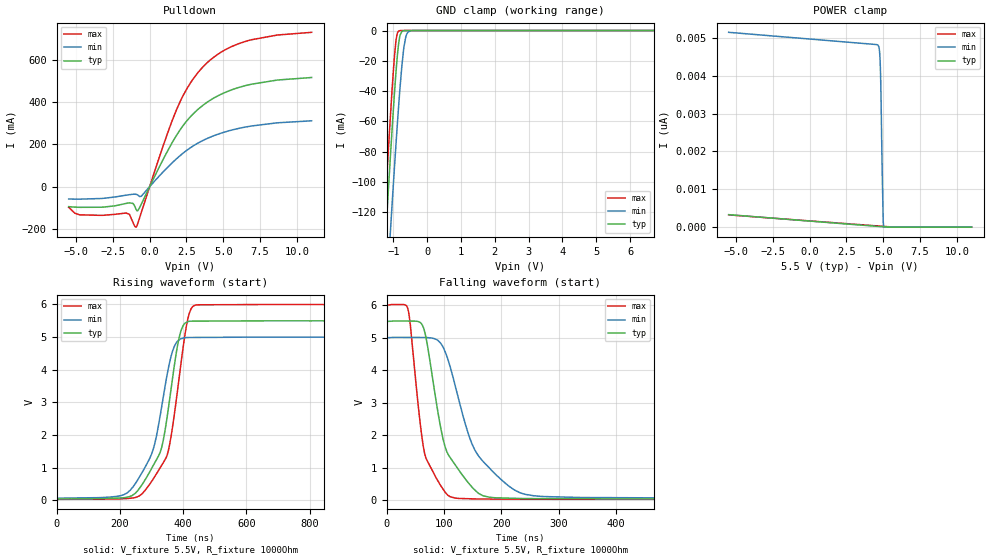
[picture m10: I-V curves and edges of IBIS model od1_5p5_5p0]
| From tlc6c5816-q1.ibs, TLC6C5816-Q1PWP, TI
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|   od1_5p5_5p0 Model
[Model]   od1_5p5_5p0
Model_type   Open_drain
Polarity   Inverting
Vmeas = 2.75
Vref = 5.5
Cref = 2pF
Rref = 1000
|   typ   min   max
C_comp   4.463pF   3.923pF   4.609pF
| Where Nom  PVT is Nominal Process, 5.5V, 27C
|   Fast PVT is Strong Process,  6.0V, -40C
|   Slow PVT is Weak Process,   5.0V, 150C
[Voltage Range]   5.5   5   6
|Junction Temperature
[Temperature Range]   27   150   -40
[Pullup Reference]   5.5   5   6
[Pulldown Reference]   0   -0   0
[Power Clamp Reference]   5.5   5   6
[GND Clamp Reference]   0   0   0
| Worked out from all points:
|   slope of the pulldown table from 0 to 0.825 V, typ, clamps not added: 7.09 ohm
|   GND clamp passes 1 mA (typ) near -0.76 V on its own axis
|   falling waveform, V_fixture 5.5V, R_fixture 1000Ohm: 20-80 % time 43.5ns typ, 63.8ns min, 26ns max; typ from 5.5 V to 0.038 V
|   rising waveform, V_fixture 5.5V, R_fixture 1000Ohm: 20-80 % time 67.2ns typ, 70.9ns min, 60.2ns max; typ from 0.038 V to 5.5 V
[Pulldown]
|   Voltage   I(typ)   I(min)   I(max)
-5.5V     -94.6mA    -58.44mA   -97.45mA
-4.741V   -97.79mA   -59.07mA   -133.2mA
-1.606V   -79.34mA   -40.37mA   -124.8mA
-1.144V   -79.15mA   -36.05mA   -167.2mA
-913mV    -108.3mA   -36.58mA   -191mA
-566.5mV  -82.74mA   -44.65mA   -122.2mA
1.677V    225.9mA    122.4mA    338.7mA
2.552V    313.6mA    173.5mA    466.2mA
3.476V    377.1mA    213.5mA    555.7mA
4.631V    429.7mA    248mA      626.5mA
6.248V    473.3mA    278.5mA    681.5mA
11V       516.5mA    311.7mA    730.3mA
[GND Clamp]
|   Voltage   I(typ)   I(min)   I(max)
-5.5V     -1.93A     -1.907A    -1.997A
-1.375V   -193.6mA   -240.8mA   -169.5mA
-1.26V    -148.7mA   -197.1mA   -123.2mA
-1.194V   -123.4mA   -172.5mA   -97.38mA
-1.078V   -80.43mA   -130.2mA   -53.97mA
-995.5mV  -51.41mA   -100.8mA   -25.95mA
-929.5mV  -30.24mA   -78.14mA   -8.512mA
-830.5mV  -6.789mA   -46.41mA   -244.4uA
-682mV    -66.71uA   -10.45mA   -495.5nA
-599.5mV  -3.753uA   -2.242mA   -28.35nA
-451mV    -21.84nA   -64.6uA    -307pA
11V       0A         0A         0A
[POWER Clamp]
|   Voltage   I(typ)   I(min)   I(max)
-5.5V     329.9pA    5.145nA    324.3pA
4.631V    20.22pA    4.807nA    31.57pA
4.73V     17.33pA    4.699nA    28.77pA
4.763V    16.38pA    4.565nA    27.84pA
4.796V    15.43pA    4.299nA    26.91pA
4.829V    14.48pA    3.819nA    25.99pA
4.846V    14.01pA    3.484nA    25.52pA
4.912V    12.14pA    1.848nA    23.67pA
4.978V    10.29pA    530.8pA    21.83pA
4.994V    9.839pA    158.8pA    21.37pA
5.027V    8.939pA    0A         20.45pA
11V       0A         0A         0A
[Ramp]
R_load = 1000
|   typ   min   max
dV/dt_r   3.2774/6.71721e-08   2.96253/7.08747e-08   3.58336/6.02096e-08
dV/dt_f   3.27744/4.34776e-08   2.96258/6.36557e-08   3.58339/2.59827e-08
[Falling Waveform]
V_fixture = 5.5V
V_fixture_min = 5V
V_fixture_max = 6V
R_fixture = 1000Ohm
C_fixture = 0F
|   Time   V(typ)   V(min)   V(max)
0s        5.5V       5V         6V
37.69ns   5.513V     5.01V      5.855V
62.54ns   5.387V     5.008V     1.851V
68.6ns    5.027V     5.007V     1.303V
98.55ns   1.886V     4.716V     341.7mV
119.2ns   1.104V     3.563V     68.31mV
159.5ns   225.1mV    1.388V     38.04mV
223.1ns   59.09mV    315mV      33.66mV
265.9ns   49.71mV    123.3mV    31.11mV
2.5us     37.6mV     62.36mV    27.69mV
[Rising Waveform]
V_fixture = 5.5V
V_fixture_min = 5V
V_fixture_max = 6V
R_fixture = 1000Ohm
C_fixture = 0F
|   Time   V(typ)   V(min)   V(max)
0s        37.6mV     62.36mV    27.69mV
213.1ns   77.87mV    172.5mV    46.9mV
288.7ns   771.1mV    1.176V     415.1mV
331.4ns   1.592V     2.825V     1.059V
350.3ns   2.606V     3.895V     1.408V
366.7ns   3.749V     4.577V     2.257V
390.1ns   5.092V     4.936V     3.961V
411.3ns   5.456V     4.987V     5.394V
439.2ns   5.49V      4.989V     5.982V
2.5us     5.5V       5V         6V
